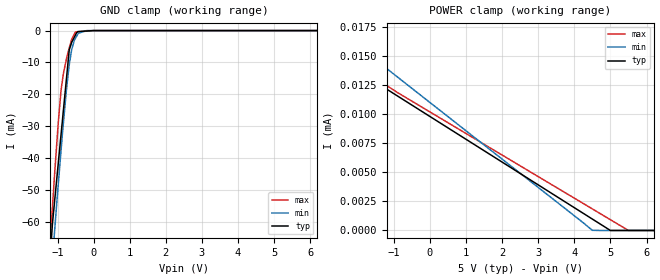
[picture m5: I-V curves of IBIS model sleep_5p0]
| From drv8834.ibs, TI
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|   sleep_5p0 Model
[Model]   sleep_5p0
Model_type   Input
Vinl = 0.7
Vinh = 2
|   typ   min   max
|   (nom PVT)   (fast PVT)   (slow PVT)
|C_comp from frequency sweep method (F=250KHz)
|Average
|C_comp   2.623e-12   2.404e-12   2.849e-12
|C_comp from LC tank measurement(L=1nH)
|Average
|Resonant Frequency(Hz)   4.390e+09   4.440e+09   4.310e+09
 C_comp   1.316e-12   1.286e-12   1.365e-12
| Where nom  PVT is Nominal Process, 5V, 27C
|   Fast PVT is Strong Process,  5.5V, -40C
|   Slow PVT is Weak Process,   4.5V, 125C
[Voltage Range]   5   4.5   5.5
|Ambient Temperature   25   150   -40
|Junction Temperature
[Temperature Range]   27   125   -40
[Power Clamp Reference]   5   4.5   5.5
[GND Clamp Reference]   0   0   0
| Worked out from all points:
|   GND clamp passes 1 mA (typ) near -0.49 V on its own axis
[GND Clamp]
|   Voltage   I(typ)   I(min)   I(max)
-5V       -796.6mA   -746.9mA   -837.8mA
-1.216V   -73.1mA    -83.06mA   -68.39mA
-1.179V   -67.02mA   -77.42mA   -62.09mA
-1.14V    -60.52mA   -71.68mA   -55.36mA
-1.078V   -53.26mA   -62.54mA   -44.66mA
-907.5mV  -33.29mA   -38.37mA   -19.47mA
-836mV    -24.91mA   -28.92mA   -13.43mA
-675mV    -6.059mA   -10.76mA   -5.498mA
-603mV    -3.586mA   -5.766mA   -2.643mA
-506mV    -1.426mA   -2.475mA   -476.3uA
-202.5mV  -140.3uA   -10.98uA   -190.6uA
10V       0A         0A         0A
[POWER Clamp]
|   Voltage   I(typ)   I(min)   I(max)
-5V       1.684mA    1.439mA    1.994mA
-1.738V   98.34uA    19.38uA    213.9uA
-1.575V   34.97uA    14.93uA    131.6uA
-1.507V   19.95uA    14.75uA    97.3uA
-1.375V   12.59uA    14.4uA     38.36uA
-1.315V   12.44uA    14.25uA    19.63uA
-1.298V   12.4uA     14.21uA    16.65uA
-1.26V    12.31uA    14.11uA    13.37uA
-1.199V   12.19uA    13.96uA    12.5uA
4.495V    991.6nA    15.32nA    1.866uA
5.495V    0A         0A         10.21nA
10V       0A         0A         0A
